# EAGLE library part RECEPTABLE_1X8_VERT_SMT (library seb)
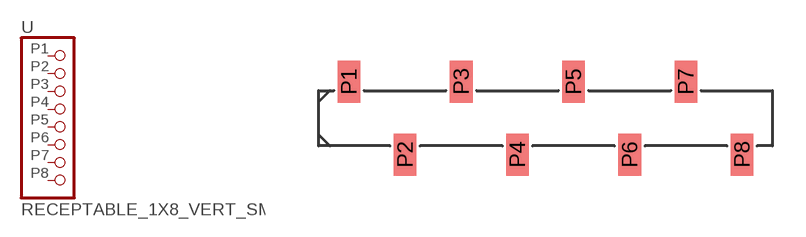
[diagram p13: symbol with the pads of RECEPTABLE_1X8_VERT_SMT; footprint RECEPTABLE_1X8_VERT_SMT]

Designator prefix -

## RECEPTABLE_1X8_VERT_SMT  [RECEPTABLE_1X8_VERT_SMT]
P1  1  pas
P2  2  pas
P3  3  pas
P4  4  pas
P5  5  pas
P6  6  pas
P7  7  pas
P8  8  pas

## Footprint RECEPTABLE_1X8_VERT_SMT (pad centres in mm)
smd 1.02 x 1.9: P1 -7.62,1.65; P2 -5.08,-1.65; P3 -2.54,1.65; P4 0,-1.65; P5 2.54,1.65; P6 5.08,-1.65; P7 7.62,1.65; P8 10.16,-1.65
